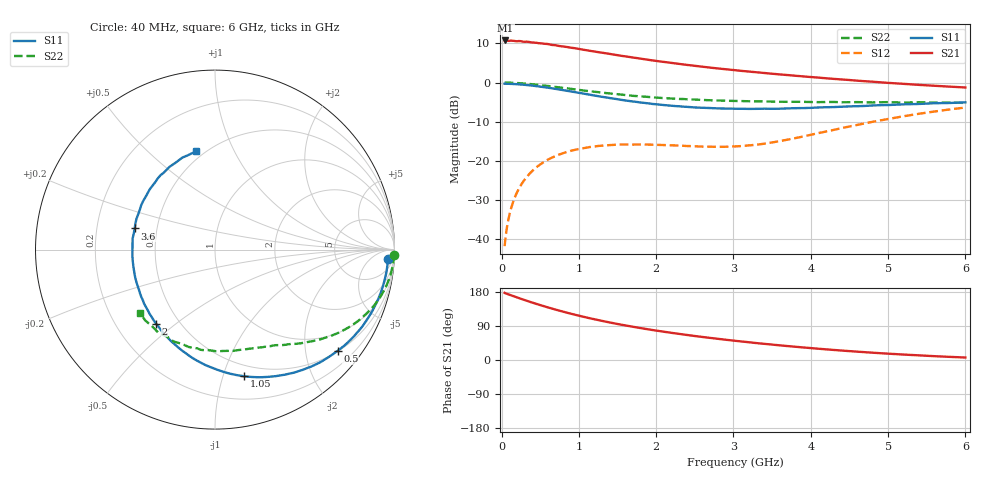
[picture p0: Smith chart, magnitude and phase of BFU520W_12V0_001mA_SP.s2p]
! Filename:  P:\Prog\Test\Noise\ATS_data\Testdata_Net\Run2\BFU520W_APM2013_06_A05_12p0V_001mA_SP_CM01_D.s2p
! Date/Time: Tue 26/Mar/2013 18:01:43
! BFU520W_APM2013_06_A05_12p0V_1to20mA_SP_CM01_Bias1_R.s2p
! MDIF S-parameter v. bias file
! BFU520W_APM2013_06_A05_12p0V_1to20mA_SP_CM01
! Date/time Thu Mar 21 16:35:01 2013
! bias mode 1
! bias variable = I_out
! VAR bias_var= 1
! VAR V_out= 12.0000
! VAR I_out= 0.9950
! VAR V_in= 0.7889
! VAR I_in= 0.0092
! Device data file deembeded for feedlines and parallel
! Original file: \Run2\BFU520W_APM2013_06_A05_12p0V_001mA_SP_CM01_R.s2p
! Feed-files: PR019V01_070313_Feed1.s2p, PR019V01_070313_Feed2.s2p
! Parallel-file: PR019V01_070313_Par.s2p
# MHz S MA R 50
!  Freq-MHz  S11-mag  S11-arg  S21-mag  S21-arg  S12-mag  S12-arg  S22-mag  S22-arg
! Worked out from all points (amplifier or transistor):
!   98 points, 40 MHz to 6 GHz, reference 50 ohm
!   highest |S21| = 10.8 dB at 50 MHz (marker M1)
!   |S21| within 3 dB of that: start of sweep to 1.255 GHz
!   unconditionally stable (mu >= 1): 2.789 GHz to 3.732 GHz
!   at 300 MHz: K = 0.12, MSG = 17.6 dB, |S12| = -24.8 dB
!   at 1.6 GHz: K = 0.57, MSG = 11.3 dB, |S12| = -15.9 dB
!   at 6 GHz: K = 0.80, MSG = 2.6 dB, |S12| = -6.4 dB
!   S11 on the Smith chart (normalised r, x): 40 MHz: 16, -25; 500 MHz: 0.51, -2.69; 1.05 GHz: 0.40, -1.18; 2 GHz: 0.37, -0.43; 3.6 GHz: 0.37, +0.11; 6 GHz: 0.45, +0.72
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40  0.9654 -3.3  3.447 177.2  0.008081 87.2  0.9982 -1.6
50  0.9655 -4.1  3.451 176.0  0.009988 86.8  0.9976 -2.1
100  0.9626 -8.2  3.407 172.4  0.01993 84.2  0.9948 -4.5
120  0.9603 -9.8  3.436 171.0  0.02384 83.2  0.9941 -5.4
200  0.9513 -16.2  3.369 165.2  0.03925 79.0  0.9851 -9.0
240  0.9444 -19.5  3.388 162.3  0.04667 77.0  0.98 -10.8
340  0.9261 -27.4  3.317 155.4  0.0643 72.0  0.962 -15.0
500  0.886 -39.6  3.178 144.9  0.08958 64.6  0.9277 -21.2
700  0.8283 -54.1  2.996 132.9  0.115 56.5  0.8783 -28.1
850  0.7825 -64.3  2.841 124.6  0.1299 51.3  0.8414 -32.6
1050  0.7247 -77.0  2.634 114.5  0.1442 45.4  0.7934 -37.8
1250  0.6695 -88.9  2.446 105.4  0.1544 40.5  0.7539 -42.2
1500  0.6116 -103.0  2.237 95.0  0.1604 35.8  0.7088 -47.4
1800  0.5555 -118.6  2.021 84.2  0.1612 32.5  0.6641 -52.6
2000  0.5272 -128.6  1.89 77.7  0.1597 31.4  0.6424 -56.0
2050  0.5215 -130.8  1.861 76.2  0.1592 31.3  0.6371 -56.7
2500  0.4799 -151.6  1.636 63.3  0.153 33.0  0.6057 -63.9
3100  0.4614 -176.5  1.41 49.0  0.154 44.0  0.5795 -74.1
3600  0.4626 165.2  1.269 38.6  0.1782 54.7  0.568 -83.4
4100  0.4799 149.0  1.156 29.7  0.2257 60.4  0.5614 -93.8
5200  0.5262 118.9  0.9621 14.4  0.3703 56.6  0.5535 -119.0
6000  0.5578 101.1  0.8641 6.5  0.4789 47.3  0.5484 -139.7
